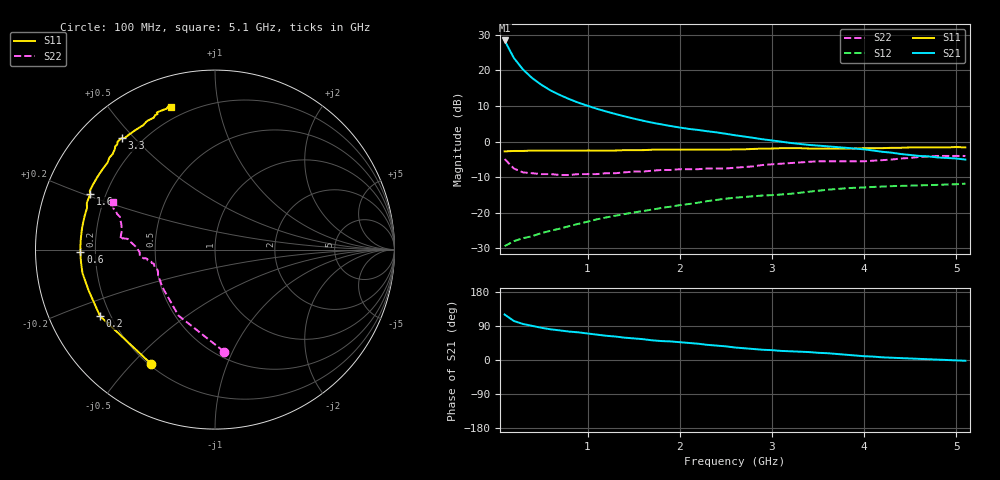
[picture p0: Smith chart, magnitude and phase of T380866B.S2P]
!AT-38086
!S-PARAMETERS at Vce=6.0V  Ic=50mA.  LAST UPDATED 08-05-96
# ghz s ma r 50
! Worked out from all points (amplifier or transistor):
!   51 points, 100 MHz to 5.1 GHz, reference 50 ohm
!   highest |S21| = 28.4 dB at 100 MHz (marker M1)
!   |S21| within 3 dB of that: start of sweep to 161.1 MHz
!   unconditionally stable (mu >= 1): 874.5 MHz to end of sweep
!   at 900 MHz: K = 1.01, MAG = 16.4 dB, |S12| = -23.1 dB
!   at 2.6 GHz: K = 1.10, MAG = 6.8 dB, |S12| = -15.8 dB
!   at 5.1 GHz: K = 1.07, MAG = 1.7 dB, |S12| = -11.8 dB
!   S11 on the Smith chart (normalised r, x): 100 MHz: 0.21, -0.57; 200 MHz: 0.16, -0.26; 600 MHz: 0.14, -0.01; 1.6 GHz: 0.14, +0.21; 3.3 GHz: 0.13, +0.46; 5.1 GHz: 0.14, +0.73
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0.1  0.73 -119.0  26.41 120.0  0.034 40.0  0.57 -85.0
0.2  0.74 -150.0  15.01 103.0  0.04 34.0  0.42 -119.0
0.3  0.74 -162.0  10.3 95.0  0.044 35.0  0.37 -136.0
0.4  0.75 -170.0  7.8 90.0  0.047 38.0  0.36 -145.0
0.5  0.75 -175.0  6.28 85.0  0.052 42.0  0.35 -151.0
0.6  0.75 -179.0  5.23 81.0  0.056 45.0  0.35 -155.0
0.7  0.75 178.0  4.52 78.0  0.06 47.0  0.34 -159.0
0.8  0.75 175.0  3.97 75.0  0.065 49.0  0.34 -161.0
0.9  0.75 172.0  3.53 73.0  0.07 51.0  0.35 -163.0
1  0.75 170.0  3.19 70.0  0.075 52.0  0.35 -165.0
1.1  0.75 167.0  2.9 67.0  0.081 53.0  0.35 -167.0
1.2  0.75 165.0  2.66 64.0  0.086 54.0  0.36 -168.0
1.4  0.76 160.0  2.27 59.0  0.096 55.0  0.37 -170.0
1.6  0.76 156.0  1.97 55.0  0.106 56.0  0.38 -172.0
1.8  0.77 153.0  1.75 50.0  0.117 56.0  0.4 -173.0
2.6  0.78 139.0  1.23 33.0  0.163 54.0  0.43 -180.0
2.9  0.8 134.0  1.08 27.0  0.175 52.0  0.47 175.0
3.3  0.81 130.0  0.93 22.0  0.191 51.0  0.51 173.0
3.5  0.8 128.0  0.88 19.0  0.204 50.0  0.53 174.0
3.9  0.8 120.0  0.8 12.0  0.225 45.0  0.53 170.0
4.3  0.82 114.0  0.7 6.0  0.237 41.0  0.56 161.0
5.1  0.83 107.0  0.56 -2.0  0.257 36.0  0.63 155.0
